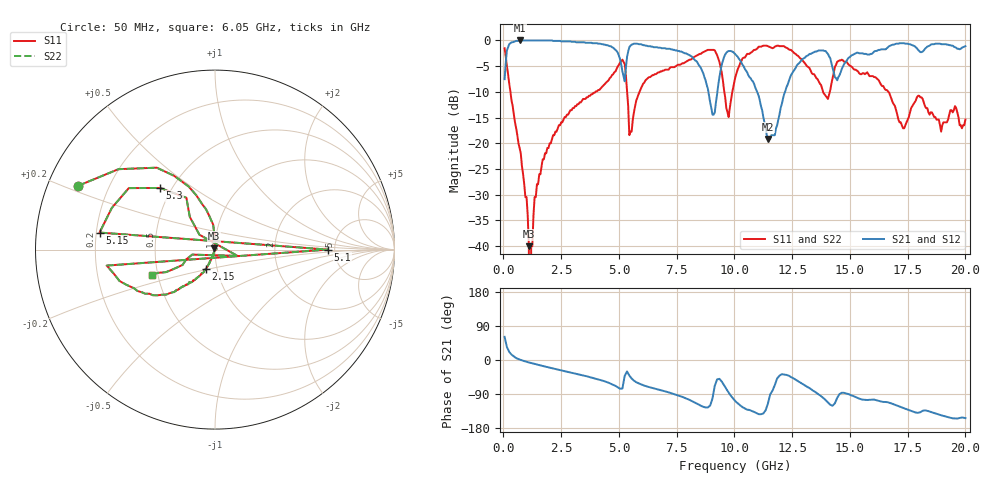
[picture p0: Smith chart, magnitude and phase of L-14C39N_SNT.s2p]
#	mhz	s	ma	r	50
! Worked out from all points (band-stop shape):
!   400 points, 50 MHz to 20 GHz, reference 50 ohm
!   highest |S21| = 0.00 dB at 700 MHz (marker M1); lowest = -19.2 dB at 11.45 GHz (marker M2)
!   |S21| within 3 dB of the highest: 127.5 MHz to 5.002 GHz (4.875 GHz wide, 190 % of centre); 15.04 GHz to end of sweep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
!   lowest |S11| = -40.0 dB at 1.1 GHz (marker M3), VSWR 1.02, Z = 49.4 + j0.784 ohm
!   |S11| at or under -10 dB: 302.9 MHz to 3.981 GHz (3.678 GHz wide, 172 % of centre); 5.356 GHz to 5.891 GHz (534.9 MHz wide, 9.51 % of centre); 16.67 GHz to end of sweep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
!   |S22| runs from - to -1.0 dB; largest |S21 - S12| = 0
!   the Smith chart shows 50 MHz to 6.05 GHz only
!   S11 on the Smith chart (normalised r, x): 50 MHz: 0.09, +0.22; 2.15 GHz: 0.88, -0.19; 5.1 GHz: 4.41, +0.00; 5.15 GHz: 0.21, +0.07; 5.3 GHz: 0.43, +0.38; 6.05 GHz: 0.46, -0.15
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50  0.84 154.9  0.42 61.1  0.42 61.1  0.84 154.9
700  0.09 91.2  1 1.2  1 1.2  0.09 91.2
1100  0.01 127.5  1 -6.4  1 -6.4  0.01 127.5
1150  0 155.0  1 -7.3  1 -7.3  0 155.0
1200  0.01 21.0  1 -8.1  1 -8.1  0.01 21.0
1350  0.03 -111.7  1 -10.4  1 -10.4  0.03 -111.7
2150  0.12 -115.2  0.99 -22.3  0.99 -22.3  0.12 -115.2
3400  0.26 -129.9  0.96 -40.2  0.96 -40.2  0.26 -129.9
5050  0.61 -171.6  0.66 -75.9  0.66 -75.9  0.61 -171.6
5100  0.63 0.0  0.58 -75.6  0.58 -75.6  0.63 0.0
5150  0.65 171.6  0.5 -75.2  0.5 -75.2  0.65 171.6
5300  0.46 131.7  0.54 -36.0  0.54 -36.0  0.46 131.7
6050  0.38 -158.5  0.9 -66.8  0.9 -66.8  0.38 -158.5
6700  0.49 -170.7  0.85 -77.8  0.85 -77.8  0.49 -170.7
7050  0.52 -178.4  0.83 -83.8  0.83 -83.8  0.52 -178.4
7100  0.52 0.6  0.83 -84.5  0.83 -84.5  0.52 0.6
7200  0.54 178.5  0.83 -86.4  0.83 -86.4  0.54 178.5
10050  0.45 154.1  0.73 -109.3  0.73 -109.3  0.45 154.1
11450  0.88 97.1  0.11 -114.9  0.11 -114.9  0.88 97.1
13350  0.48 41.1  0.75 -78.8  0.75 -78.8  0.48 41.1
16700  0.31 -14.2  0.88 -112.6  0.88 -112.6  0.31 -14.2
20000  0.17 -76.7  0.88 -153.3  0.88 -153.3  0.17 -76.7
